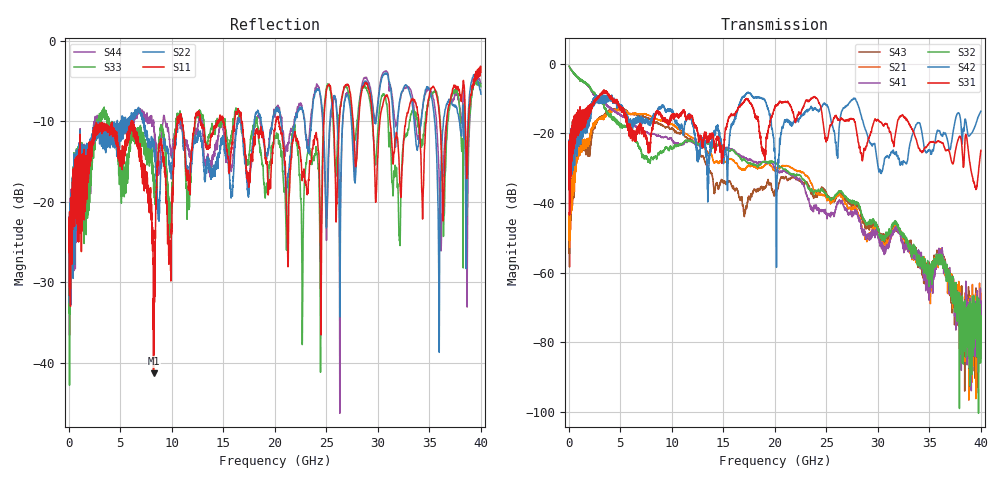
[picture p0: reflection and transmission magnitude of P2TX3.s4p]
!Agilent Technologies,N5245A,MY49151084,A.09.20.08
!Agilent N5245A: A.09.20.08
!Date: Thursday, March 01, 2012 10:47:45
!Correction: S11(Full 4 Port(1,2,3,4))
!S12(Full 4 Port(1,2,3,4))
!S13(Full 4 Port(1,2,3,4))
!S14(Full 4 Port(1,2,3,4))
!S21(Full 4 Port(1,2,3,4))
!S22(Full 4 Port(1,2,3,4))
!S23(Full 4 Port(1,2,3,4))
!S24(Full 4 Port(1,2,3,4))
!S31(Full 4 Port(1,2,3,4))
!S32(Full 4 Port(1,2,3,4))
!S33(Full 4 Port(1,2,3,4))
!S34(Full 4 Port(1,2,3,4))
!S41(Full 4 Port(1,2,3,4))
!S42(Full 4 Port(1,2,3,4))
!S43(Full 4 Port(1,2,3,4))
!S44(Full 4 Port(1,2,3,4))
!S4P File: Measurements: <S11,S12,S13,S14>,
!<S21,S22,S23,S24>,
!<S31,S32,S33,S34>,
!<S41,S42,S43,S44>:
# Hz S  dB  R 50
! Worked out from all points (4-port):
!   3996 points, 50 MHz to 40 GHz, reference 50 ohm
!   strongest paths, dB at 50 MHz, 10.04 GHz, 20.03 GHz, 30.02 GHz, 40 GHz:
!     S31: -25.6, -15.2, -12.3, -16.2, -24.9
!     S42: -24.6, -13.3, -27.2, -29.4, -13.7
!     S32: -0.7, -24.6, -28.5, -47.6, -81.7
!     S41: -0.8, -21.9, -30.0, -49.1, -68.2
!     S21: -44.3, -17.4, -30.5, -48.2, -84.5
!     S43: -45.2, -18.6, -36.5, -47.2, -72.4
!   lowest |S11| = -41.3 dB at 8.24 GHz (marker M1), VSWR 1.02, Z = 49.6 + j0.772 ohm
!   |S11| at or under -10 dB: start of sweep to 6.099 GHz; 6.17 GHz to 10.55 GHz (4.376 GHz wide, 52.4 % of centre); 20.37 GHz to 24.77 GHz (4.398 GHz wide, 19.5 % of centre)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
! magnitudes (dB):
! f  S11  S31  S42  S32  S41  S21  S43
! 50 MHz  -23.0  -25.6  -24.6  -0.7  -0.8  -44.3  -45.2
! 2.88 GHz  -10.6  -9.7  -9.4  -10.1  -10.0  -15.9  -15.9
! 8.24 GHz  -41.3  -17.3  -15.0  -27.3  -20.2  -15.5  -16.8
! 18.78 GHz  -11.7  -24.9  -10.0  -28.3  -28.3  -29.8  -35.8
! 20.22 GHz  -9.6  -12.0  -34.1  -28.9  -31.0  -29.9  -36.4
! 26.45 GHz  -7.6  -15.6  -14.0  -36.8  -39.7  -37.8  -37.2
! 40 GHz  -3.9  -24.9  -13.7  -81.7  -68.2  -84.5  -72.4
